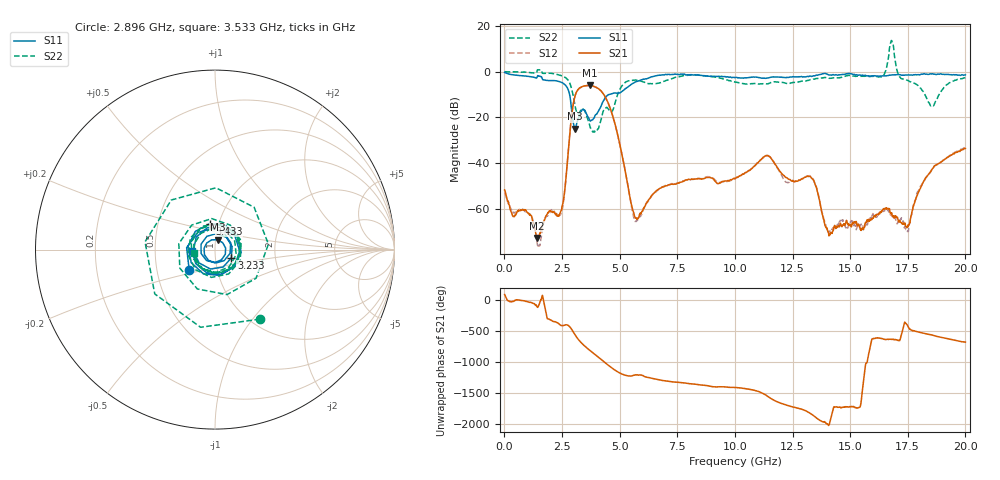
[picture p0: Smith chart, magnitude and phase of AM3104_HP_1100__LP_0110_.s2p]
!Created with skrf (http://scikit-rf.org).
# Hz S RI R 50.0
!freq ReS11 ImS11 ReS21 ImS21 ReS12 ImS12 ReS22 ImS22
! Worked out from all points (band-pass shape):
!   1601 points, 10 MHz to 20 GHz, reference 50 ohm
!   highest |S21| = -6.02 dB at 3.696 GHz (marker M1); lowest = -72.5 dB at 1.397 GHz (marker M2)
!   |S21| within 3 dB of the highest: 3.122 GHz to 4.241 GHz (1.119 GHz wide, 30.4 % of centre)
!   lowest |S11| = -24.9 dB at 3.071 GHz (marker M3), VSWR 1.12, Z = 51.2 + j5.65 ohm
!   |S11| at or under -10 dB: 2.829 GHz to 4.54 GHz (1.711 GHz wide, 46.5 % of centre)
!   |S22| runs from -26.4 to 13.6 dB; largest |S21 - S12| = 0.029
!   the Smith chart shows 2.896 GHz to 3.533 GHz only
!   S11 on the Smith chart (normalised r, x): 2.896 GHz: 0.73, -0.17; 3.233 GHz: 1.20, -0.11; 3.433 GHz: 0.91, +0.27; 3.533 GHz: 0.77, -0.01
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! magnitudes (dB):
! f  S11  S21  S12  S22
! 10 MHz  -0.4  -51.6  -53.0  0.0
! 1.397 GHz  -2.8  -72.5  -73.4  -0.5
! 2.471 GHz  -4.7  -60.5  -61.7  -1.8
! 2.896 GHz  -14.8  -21.2  -21.3  -6.7
! 3.071 GHz  -24.9  -10.4  -10.4  -15.2
! 3.233 GHz  -19.8  -7.4  -7.5  -18.3
! 3.346 GHz  -17.2  -6.7  -6.8  -16.5
! 3.433 GHz  -16.6  -6.3  -6.4  -16.6
! 3.533 GHz  -17.8  -6.1  -6.2  -18.4
! 3.696 GHz  -21.0  -6.0  -6.1  -23.2
! 4.62 GHz  -9.7  -16.7  -16.9  -17.5
! 5.67 GHz  -4.6  -63.6  -65.4  -3.7
! 6.682 GHz  -1.6  -51.4  -51.4  -5.1
! 10.01 GHz  -2.7  -46.7  -46.6  -4.6
! 11.39 GHz  -2.9  -36.6  -36.8  -5.3
! 13.34 GHz  -2.1  -46.6  -46.3  -3.5
! 14.12 GHz  -1.5  -71.3  -69.6  -2.9
! 16.36 GHz  -1.9  -61.1  -61.0  -2.3
! 16.68 GHz  -1.6  -59.9  -61.3  7.1
! 17.48 GHz  -1.5  -67.8  -69.7  -3.8
! 18.54 GHz  -1.0  -42.8  -42.8  -14.7
! 20 GHz  -1.4  -33.5  -32.9  -2.7
